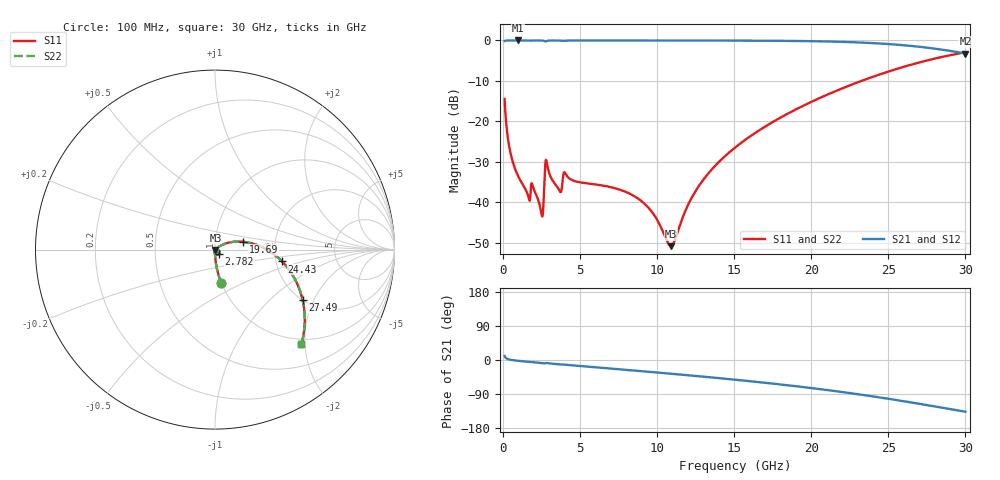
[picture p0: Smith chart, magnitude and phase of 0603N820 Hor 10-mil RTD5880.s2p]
# GHz S MA R 50
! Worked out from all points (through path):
!   3201 points, 100 MHz to 30 GHz, reference 50 ohm
!   highest |S21| = -0.01 dB at 940.9 MHz (marker M1); lowest = -3.2 dB at 30 GHz (marker M2)
!   group delay of S21, straight-line fit = 12.2 ps
!   lowest |S11| = -50.9 dB at 10.88 GHz (marker M3), VSWR 1.01, Z = 50.2 - j0.177 ohm
!   |S11| at or under -10 dB: start of sweep to 23.26 GHz
!   |S22| runs from -50.9 to -2.9 dB; largest |S21 - S12| = 0
!   S11 on the Smith chart (normalised r, x): 100 MHz: 1.00, -0.38; 2.782 GHz: 1.04, -0.05; 19.69 GHz: 1.37, +0.12; 24.43 GHz: 2.16, -0.33; 27.49 GHz: 2.00, -1.65; 30 GHz: 0.90, -1.93
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0.1  0.1887 -79.4  0.9817 10.5  0.9817 10.5  0.1887 -79.4
0.4457187  0.04375 -88.4  0.9985 1.0  0.9985 1.0  0.04375 -88.4
0.9409375  0.02175 -90.0  0.999 -1.9  0.999 -1.9  0.02175 -90.0
1.623031  0.01203 -86.9  0.9982 -4.8  0.9982 -4.8  0.01203 -86.9
1.96875  0.01493 -85.7  0.9972 -5.8  0.9972 -5.8  0.01493 -85.7
2.473313  0.007489 -70.8  0.9965 -8.0  0.9965 -8.0  0.007489 -70.8
2.56675  0.006858 -37.9  0.994 -8.5  0.994 -8.5  0.006858 -37.9
2.781656  0.03339 -49.0  0.9745 -8.2  0.9745 -8.2  0.03339 -49.0
3.659969  0.01388 -85.9  0.9961 -11.6  0.9961 -11.6  0.01388 -85.9
4.033719  0.02275 -86.7  0.9936 -12.4  0.9936 -12.4  0.02275 -86.7
5.089563  0.01747 -99.6  0.9978 -16.2  0.9978 -16.2  0.01747 -99.6
8.285125  0.01254 -106.2  0.9974 -27.0  0.9974 -27.0  0.01254 -106.2
10.06978  0.005708 -95.1  0.9972 -33.3  0.9972 -33.3  0.005708 -95.1
10.88269  0.002857 -38.1  0.997 -36.2  0.997 -36.2  0.002857 -38.1
12.64866  0.01528 35.1  0.9965 -42.6  0.9965 -42.6  0.01528 35.1
15.05  0.04726 33.3  0.9948 -51.9  0.9948 -51.9  0.04726 33.3
19.69384  0.163 15.5  0.9807 -72.5  0.9807 -72.5  0.163 15.5
20.03956  0.1752 13.9  0.9784 -74.2  0.9784 -74.2  0.1752 13.9
24.43113  0.3792 -10.0  0.9166 -98.7  0.9166 -98.7  0.3792 -10.0
25.01978  0.413 -13.6  0.9016 -102.4  0.9016 -102.4  0.413 -13.6
27.48653  0.5636 -29.9  0.8151 -118.9  0.8151 -118.9  0.5636 -29.9
30  0.7132 -47.5  0.6881 -136.5  0.6881 -136.5  0.7132 -47.5
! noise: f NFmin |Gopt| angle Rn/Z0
0.1  0.0002795  0.9149  0.3823  0.000724
3.417  0.004391  0.8243  11.57  0.005196
6.743  0.005588  0.7424  22.7  0.004187
10.06  0.007636  0.7258  33.53  0.005084
13.39  0.009866  0.7238  44.02  0.006118
16.7  0.0124  0.7312  54.05  0.007341
20.03  0.01545  0.7459  63.64  0.008896
23.35  0.01928  0.7667  72.75  0.011
26.67  0.02438  0.7926  81.48  0.01407
30  0.0316  0.8227  89.85  0.01894
